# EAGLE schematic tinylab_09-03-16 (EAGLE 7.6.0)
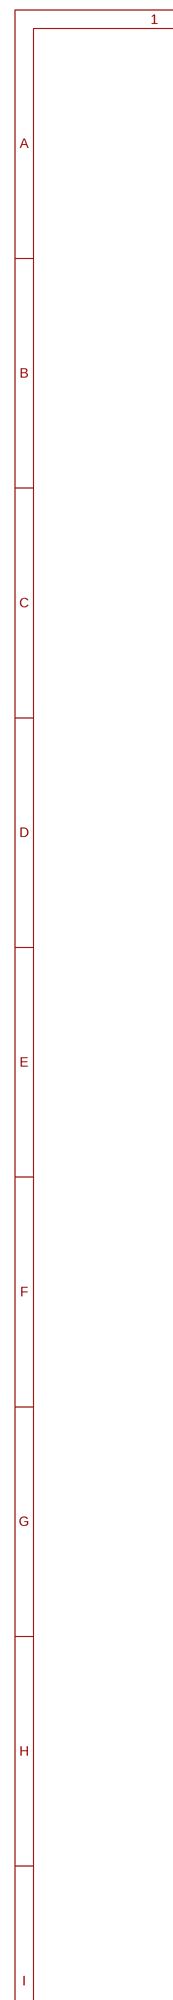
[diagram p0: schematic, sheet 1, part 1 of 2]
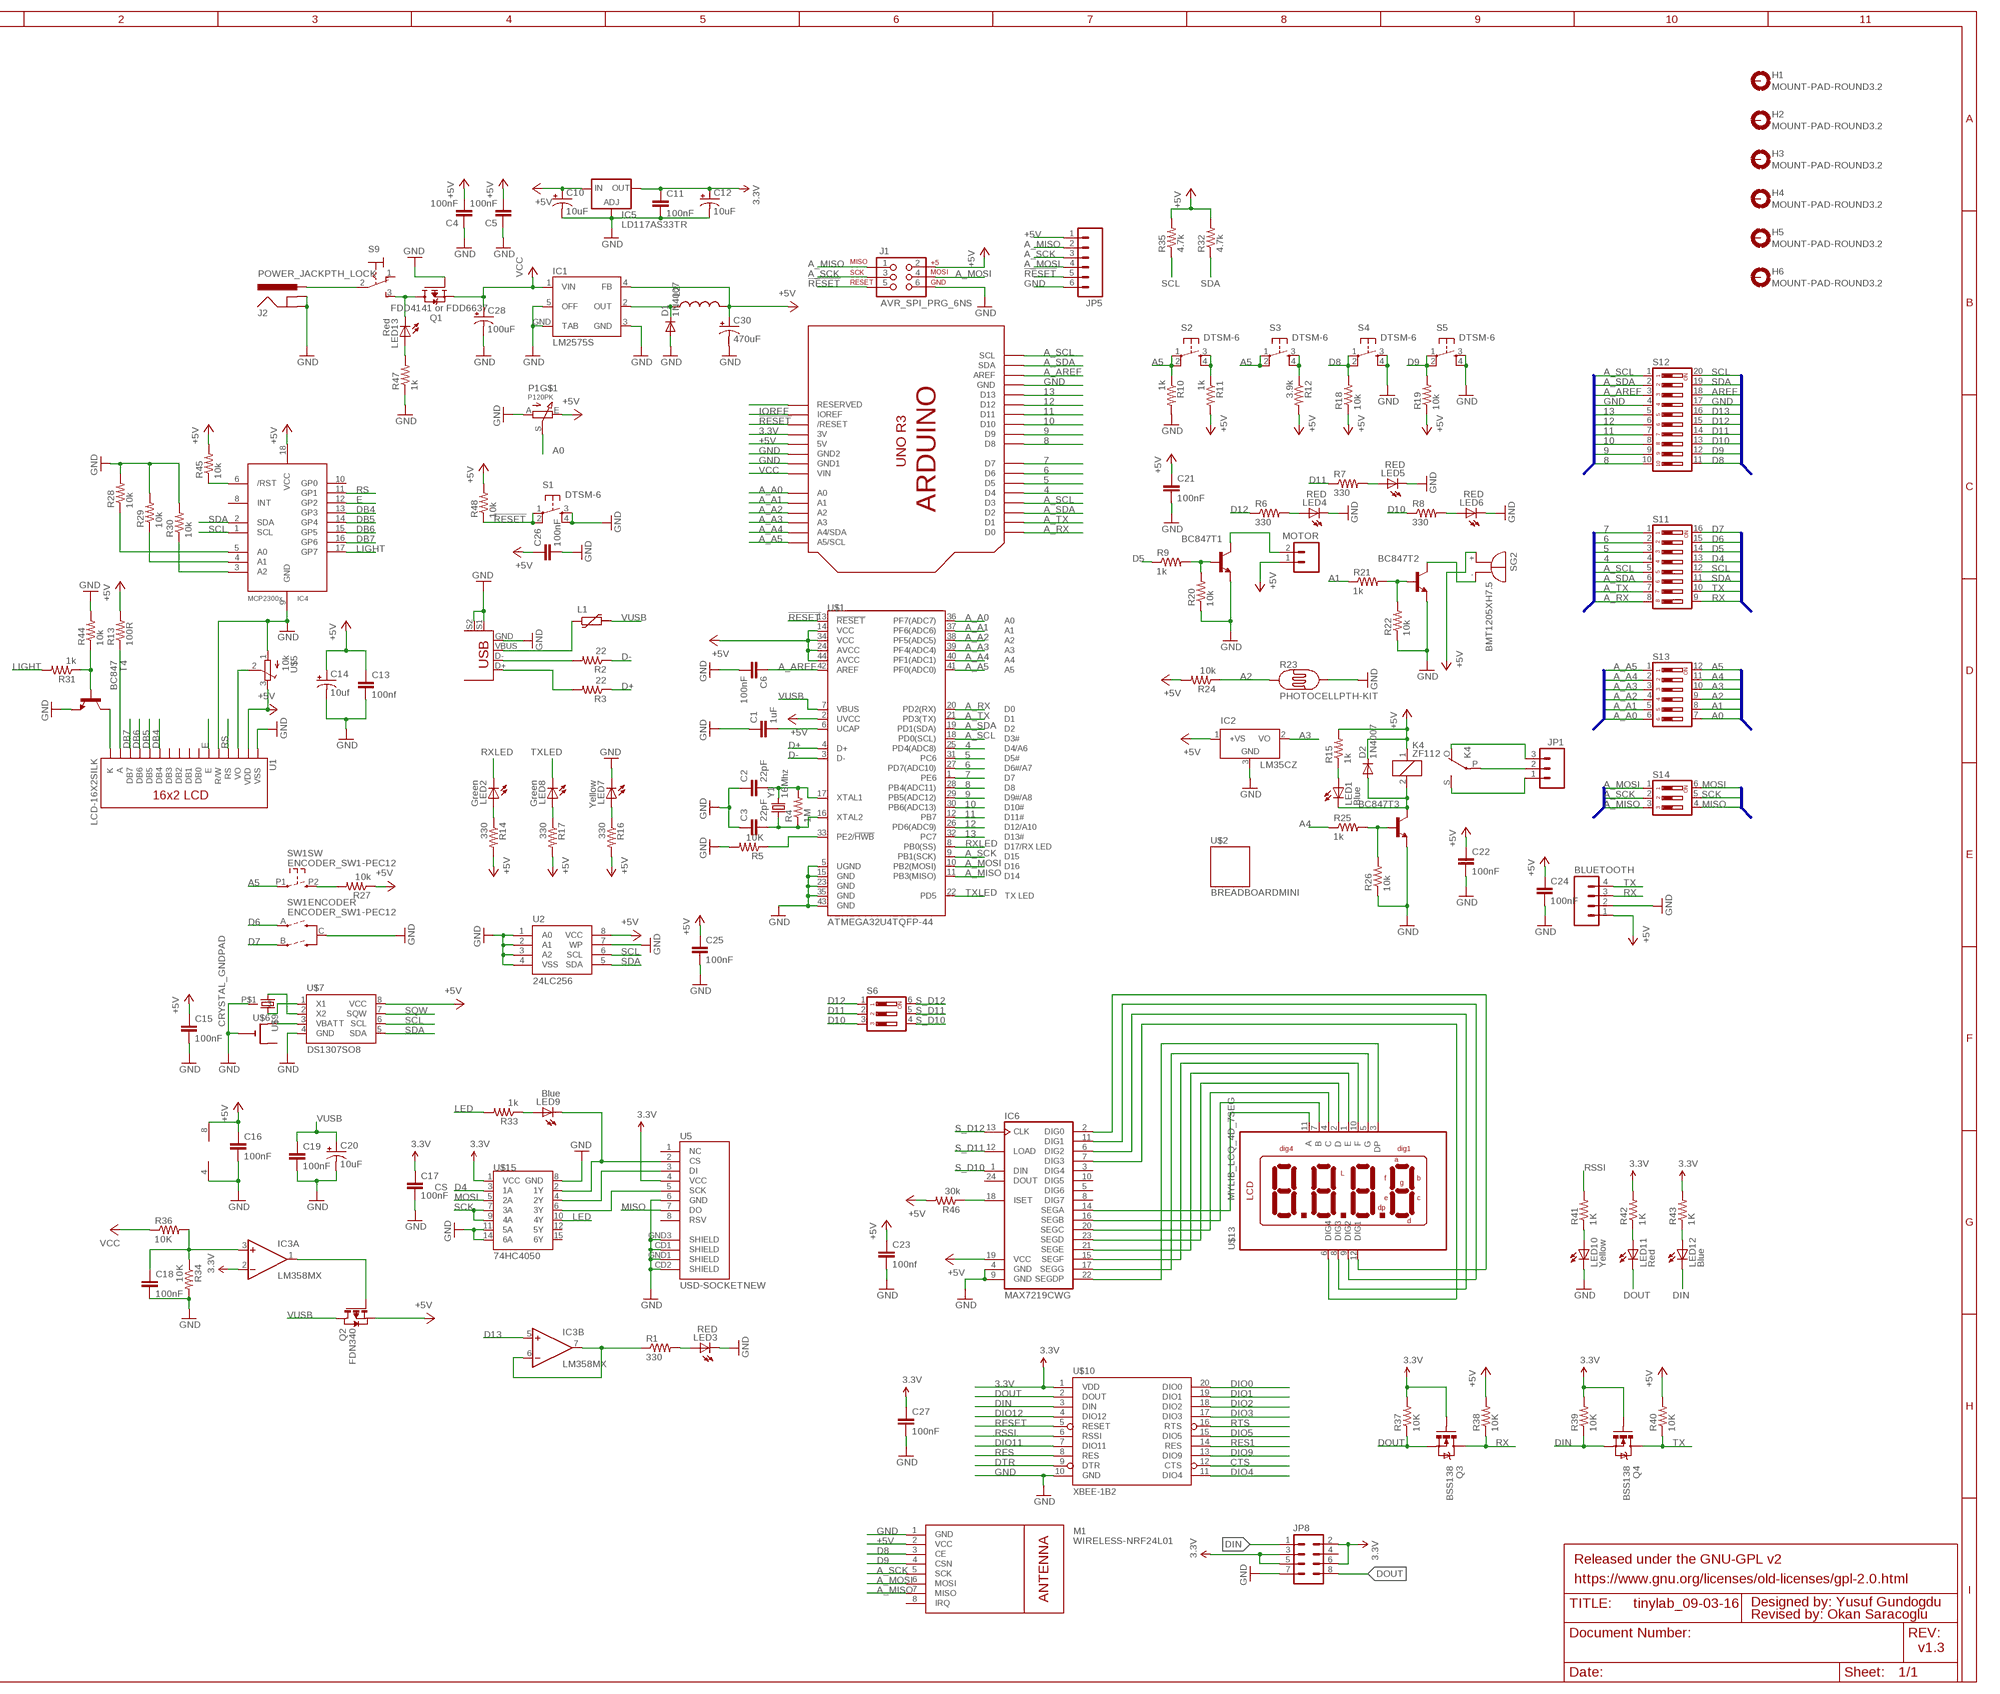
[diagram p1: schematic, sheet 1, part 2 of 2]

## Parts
BLUETOOTH  M04PTH  [1X04]
C1  1uF  CAP1206  [1206]
C2  22pF  CAP0805  [0805]
C3  22pF  CAP0805  [0805]
C4  100nF  CAP0805  [0805]
C5  100nF  CAP0805  [0805]
C6  100nF  CAP0805  [0805]
C10  10uF  CAP_POL1206  [EIA3216]
C11  100nF  CAP0805  [0805]
C12  10uF  CAP_POL1206  [EIA3216]
C13  100nf  CAP0805  [0805]
C14  10uf  CAP_POL1206  [EIA3216]
C15  100nF  CAP0805  [0805]
C16  100nF  CAP0805  [0805]
C17  100nF  CAP0805  [0805]
C18  100nF  CAP0805  [0805]
C19  100nF  CAP0805  [0805]
C20  10uF  CAP_POL1206  [EIA3216]
C21  100nF  CAP0805  [0805]
C22  100nF  CAP0805  [0805]
C23  100nf  CAP0805  [0805]
C24  100nF  CAP0805  [0805]
C25  100nF  CAP0805  [0805]
C26  100nF  CAP0805  [0805]
C27  100nF  CAP0805  [0805]
C28  100uF  CAP_POLF80  [NIPPON_F80]
C30  470uF  CAP_POLG  [PANASONIC_G]
D1  1N4007  DIODESMA-ALT  [SMA-DIODE_ALT]
D2  1N4007  DIODESMA-ALT  [SMA-DIODE_ALT]
H1  MOUNT-PAD-ROUND3.2  [3,2-PAD]
H2  MOUNT-PAD-ROUND3.2  [3,2-PAD]
H3  MOUNT-PAD-ROUND3.2  [3,2-PAD]
H4  MOUNT-PAD-ROUND3.2  [3,2-PAD]
H5  MOUNT-PAD-ROUND3.2  [3,2-PAD]
H6  MOUNT-PAD-ROUND3.2  [3,2-PAD]
IC1  LM2575S  [TO263-5]
IC2  LM35CZ  [TO92]
IC3  LM358MX  [SO08]
IC4  MCP2300X/SO  [SO18W]
IC5  LD117AS33TR  [SOT223]
IC6  MAX7219CWG  [SO24W]
J1  AVR_SPI_PRG_6NS  [2X3-NS]
J2  POWER_JACKPTH_LOCK  [POWER_JACK_PTH_LOCK]
JP1  M03-SCREW-5MM  [SCREWTERMINAL-5MM-3]
JP5  M06SIP  [1X06]
JP8  M04X2  [2X4]
K4  ZF112  [ZF112]
L1  FUSE_PTC-0805  [PTC0805]
L2  INDUCTORPWR  [CDRH125]
LED1  Blue  LEDCHIPLED_0805  [CHIPLED_0805]
LED2  Green  LEDCHIPLED_0805  [CHIPLED_0805]
LED3  RED  LED5MM  [LED5MM]
LED4  RED  LED5MM  [LED5MM]
LED5  RED  LED5MM  [LED5MM]
LED6  RED  LED5MM  [LED5MM]
LED7  Yellow  LEDCHIPLED_0805  [CHIPLED_0805]
LED8  Green  LEDCHIPLED_0805  [CHIPLED_0805]
LED9  Blue  LEDCHIPLED_0805  [CHIPLED_0805]
LED10  Yellow  LEDCHIPLED_0805  [CHIPLED_0805]
LED11  Red  LEDCHIPLED_0805  [CHIPLED_0805]
LED12  Blue  LEDCHIPLED_0805  [CHIPLED_0805]
LED13  Red  LEDCHIPLED_0805  [CHIPLED_0805]
M1  WIRELESS-NRF24L01  [WIRELESS-NRF24L01]
MOTOR  M025MM  [SCREWTERMINAL-5MM-2]
P1  P120PK  [P120PK]
Q1  FDD4141 or FDD6637  FDD4141TO252  [TO252]
Q2  FDN340  PMOSSOT23  [SOT-23]
Q3  BSS138  MOSFET-NCHANNELSMD  [SOT23-3]
Q4  BSS138  MOSFET-NCHANNELSMD  [SOT23-3]
R1  330  RESISTOR0805-RES  [0805]
R2  22  RESISTOR0805-RES  [0805]
R3  22  RESISTOR0805-RES  [0805]
R4  1M  RESISTOR0805-RES  [0805]
R5  10K  RESISTOR0805-RES  [0805]
R6  330  RESISTOR0805-RES  [0805]
R7  330  RESISTOR0805-RES  [0805]
R8  330  RESISTOR0805-RES  [0805]
R9  1k  RESISTOR0805-RES  [0805]
R10  1k  RESISTOR0805-RES  [0805]
R11  1k  RESISTOR0805-RES  [0805]
R12  3.9k  RESISTOR0805-RES  [0805]
R13  100R  RESISTOR0805-RES  [0805]
R14  330  RESISTOR0805-RES  [0805]
R15  1k  RESISTOR0805-RES  [0805]
R16  330  RESISTOR0805-RES  [0805]
R17  330  RESISTOR0805-RES  [0805]
R18  10k  RESISTOR0805-RES  [0805]
R19  10k  RESISTOR0805-RES  [0805]
R20  10k  RESISTOR0805-RES  [0805]
R21  1k  RESISTOR0805-RES  [0805]
R22  10k  RESISTOR0805-RES  [0805]
R23  PHOTOCELLPTH-KIT  [PHOTOCELL-KIT]
R24  10k  RESISTOR0805-RES  [0805]
R25  1k  RESISTOR0805-RES  [0805]
R26  10k  RESISTOR0805-RES  [0805]
R27  10k  RESISTOR0805-RES  [0805]
R28  10k  RESISTOR0805-RES  [0805]
R29  10k  RESISTOR0805-RES  [0805]
R30  10k  RESISTOR0805-RES  [0805]
R31  1k  RESISTOR0805-RES  [0805]
R32  4.7k  RESISTOR0805-RES  [0805]
R33  1k  RESISTOR0805-RES  [0805]
R34  10K  RESISTOR0805-RES  [0805]
R35  4.7k  RESISTOR0805-RES  [0805]
R36  10K  RESISTOR0805-RES  [0805]
R37  10K  RESISTOR0805-RES  [0805]
R38  10K  RESISTOR0805-RES  [0805]
R39  10K  RESISTOR0805-RES  [0805]
R40  10K  RESISTOR0805-RES  [0805]
R41  1K  RESISTOR0805-RES  [0805]
R42  1K  RESISTOR0805-RES  [0805]
R43  1K  RESISTOR0805-RES  [0805]
R44  10k  RESISTOR0805-RES  [0805]
R45  10k  RESISTOR0805-RES  [0805]
R46  30k  RESISTOR0805-RES  [0805]
R47  1k  RESISTOR0805-RES  [0805]
R48  10k  RESISTOR0805-RES  [0805]
S1  DTSM-6  [DTSM-6]
S2  DTSM-6  [DTSM-6]
S3  DTSM-6  [DTSM-6]
S4  DTSM-6  [DTSM-6]
S5  DTSM-6  [DTSM-6]
S6  DIP03YL  [DIP03YL]
S9  M9040P  [M9040P]
S11  DIP08YL  [DIP08YL]
S12  DIP10YL  [DIP10YL]
S13  DIP06YL  [DIP06YL]
S14  DIP03YL  [DIP03YL]
SG2  BMT1205XH7.5  [BMT1205XH7.5]
SW1  ENCODER_SW1-PEC12  [PEC12_INCREMENTAL_ENCODER]
T1  BC847  MMBT2222ALT1-NPN-SOT23-BEC  [SOT23-BEC]
T2  BC847  MMBT2222ALT1-NPN-SOT23-BEC  [SOT23-BEC]
T3  BC847  MMBT2222ALT1-NPN-SOT23-BEC  [SOT23-BEC]
T4  BC847  MMBT2222ALT1-NPN-SOT23-BEC  [SOT23-BEC]
U1  LCD-16X2SILK  [LCD-16X2]
U2  24LC256  EEPROM-I2CSMD  [SO08]
U5  USD-SOCKETNEW  [MICRO-SD-SOCKET-PP]
U$1  ATMEGA32U4TQFP-44  [TQFP44]
U$2  BREADBOARDMINI  [BREADBOARD-MINI]
U$3  USB+SHIELD  [USB-B-PTH]
U$4  UNO_R3  [UNO_R3]
U$5  10k  TRIMPOTTC33X  [TC33X]
U$6  CR1220SMT  [CR1220-SMD]
U$7  DS1307SO8  [SO08]
U$9  CRYSTAL_GNDPAD  [TC38H_GNDPAD]
U$10  XBEE-1B2  [XBEE-SILK]
U$13  MYLIB_LCQ_4D_7SEG  [MYLIB_LDQ_4D_7SEG]
U$15  74HC4050  HEX_CONVERTER  [SO016]
Y1  16Mhz  CRYSTAL5X3  [CRYSTAL-SMD-5X3]

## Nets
3.3V: C11.1 C12.A(+) C17.1 C27.1 IC3.2(A:-IN) IC5.4(OUT) JP8.2 JP8.3 JP8.5 JP8.6 Q3.1(G) Q4.1(G) R37.2 R39.2 R42.2 R43.2 U5.4(VCC) U$4.3V U$10.1(VDD) U$15.1(VCC)
4: S11.4 U$1.25(PD4(ADC8)) U$4.D4
5: S11.3 U$1.31(PC6) U$4.D5
6: S11.2 U$1.27(PD7(ADC10)) U$4.D6
7: S11.1 U$1.1(PE6) U$4.D7
8: S12.10 U$1.28(PB4(ADC11)) U$4.D8
9: S12.9 U$1.29(PB5(ADC12)) U$4.D9
10: S12.8 U$1.30(PB6(ADC13)) U$4.D10
11: S12.7 U$1.12(PB7) U$4.D11
12: S12.6 U$1.26(PD6(ADC9)) U$4.D12
13: S12.5 U$1.32(PC7) U$4.D13
!RESET: J1.5 JP5.5 R48.1 S1.1 S1.2 U$1.13(!RESET) U$4.RESET(/RESET)
+5V: BLUETOOTH.1 C4.2 C5.2 C10.A(+) C13.1 C14.A(+) C15.1 C16.1 C21.1 C22.1 C23.1 C24.1 C25.1 C26.1 C30.+ D2.C IC1.4(FB) IC2.1(+VS) IC3.8(P:V+) IC4.18(VCC) IC5.3(IN) IC6.19(VCC) J1.2 JP5.1 K4.1 L2.2 M1.2(VCC) MOTOR.1 P1.E Q2.2(S) R11.2 R12.2 R13.2 R14.2 R15.2 R16.2 R17.2 R18.1 R19.1 R24.2 R27.1 R32.2 R35.2 R38.2 R40.2 R45.2 R46.2 R48.2 SG2.+ U1.2(VDD) U2.8(VCC) U$1.2(UVCC) U$1.14(VCC) U$1.24(AVCC) U$1.34(VCC) U$1.44(AVCC) U$4.5V U$5.3(E) U$7.8(VCC)
A0: P1.S S13.7
A1: R21.1 S13.8
A2: R23.1 R24.1 S13.9
A3: IC2.2(VO) S13.10
A4: R25.1 S13.11
A5: R10.1 S2.1 S2.2 S3.1 S3.2 S13.12 SW1.P1
A_A0: S13.6 U$1.36(PF7(ADC7)) U$4.A0
A_A1: S13.5 U$1.37(PF6(ADC6)) U$4.A1
A_A2: S13.4 U$1.38(PF5(ADC5)) U$4.A2
A_A3: S13.3 U$1.39(PF4(ADC4)) U$4.A3
A_A4: S13.2 U$1.40(PF1(ADC1)) U$4.A4(A4/SDA)
A_A5: S13.1 U$1.41(PF0(ADC0)) U$4.A5(A5/SCL)
A_AREF: C6.1 S12.3 U$1.42(AREF) U$4.AREF
A_MISO: J1.1 JP5.2 M1.7(MISO) S14.3 U$1.11(PB3(MISO))
A_MOSI: J1.4 JP5.4 M1.6(MOSI) S14.1 U$1.10(PB2(MOSI))
A_RX: S11.8 U$1.20(PD2(RX)) U$4.D0
A_SCK: J1.3 JP5.3 M1.5(SCK) S14.2 U$1.9(PB1(SCK))
A_SCL: S11.5 S12.1 U$1.18(PD0(SCL)) U$4.D3 U$4.SCL
A_SDA: S11.6 S12.2 U$1.19(PD1(SDA)) U$4.D2 U$4.SDA
A_TX: S11.7 U$1.21(PD3(TX)) U$4.D1
AREF: S12.18
CTS: U$10.12(CTS)
D4: S11.13 U$15.3(1A)
D5: R9.1 S11.14
D6: S11.15 SW1.A(ENCODER:A)
D7: S11.16 SW1.B(ENCODER:B)
D8: M1.3(CE) R18.2 S4.1 S4.2 S12.11
D9: M1.4(CSN) R19.2 S5.1 S5.2 S12.12
D10: R8.1 S6.3 S12.13
D11: R7.1 S6.2 S12.14
D12: R6.1 S6.1 S12.15
D13: IC3.5(B:+IN) S12.16
D+: R3.1 U$1.4(D+)
D-: R2.1 U$1.3(D-)
DB4: IC4.13(GP3) U1.11(DB4)
DB5: IC4.14(GP4) U1.12(DB5)
DB6: IC4.15(GP5) U1.13(DB6)
DB7: IC4.16(GP6) U1.14(DB7)
DIN: JP8.1 LED12.C Q4.2(S) R39.1 U$10.3(DIN)
DIO0: U$10.20(DIO0)
DIO1: U$10.19(DIO1)
DIO2: U$10.18(DIO2)
DIO3: U$10.17(DIO3)
DIO4: U$10.11(DIO4)
DIO5: U$10.15(DIO5)
DIO9: U$10.13(DIO9)
DIO11: U$10.7(DIO11)
DIO12: U$10.4(DIO12)
DOUT: JP8.8 LED11.C Q3.2(S) R37.1 U$10.2(DOUT)
DTR: U$10.9(DTR)
E: IC4.12(GP2) U1.6(E)
GND: BLUETOOTH.2 C1.1 C2.1 C3.1 C4.1 C5.1 C6.2 C10.C(-) C11.2 C12.C(-) C13.2 C14.C(-) C15.2 C16.2 C17.2 C18.2 C19.2 C20.C(-) C21.2 C22.2 C23.2 C24.2 C25.2 C26.2 C27.2 C28.- C30.- D1.A IC1.3(GND) IC1.5(OFF) IC1.GND(TAB) IC2.3(GND) IC3.4(P:V-) IC4.9(GND) IC5.1(ADJ) IC6.4(GND) IC6.9(GND) J1.6 J2.GND J2.GNDBREAK JP5.6 JP8.7 LED3.K(C) LED4.K(C) LED5.K(C) LED6.K(C) LED7.C LED10.C M1.1(GND) P1.A Q1.1(G) R5.2 R10.2 R20.1 R22.1 R23.2 R26.1 R28.2 R29.2 R30.2 R34.2 R44.2 R47.1 S1.3 S1.4 S4.3 S4.4 S5.3 S5.4 S12.4 S12.17 SW1.C(ENCODER:C) T1.E T2.E T3.E T4.E U1.1(VSS) U1.5(R/W) U2.1(A0) U2.2(A1) U2.3(A2) U2.4(VSS) U2.7(WP) U5.6(GND) U5.CD1(SHIELD) U5.CD2(SHIELD) U5.GND1(SHIELD) U5.GND3(SHIELD) U$1.5(UGND) U$1.15(GND) U$1.23(GND) U$1.35(GND) U$1.43(GND) U$3.GND U$3.S1 U$3.S2 U$4.GND U$4.GND1 U$4.GND2 U$5.1(A) U$6.- U$7.4(GND) U$9.P$1 U$10.10(GND) U$15.8(GND) U$15.11(5A) U$15.14(6A)
IOREF: U$4.IOREF
LED: R33.2 U$15.10(4Y)
LIGHT: IC4.17(GP7) R31.2
MISO: S14.4 U5.7(DO)
MOSI: S14.6 U$15.5(2A)
N$1: R2.2 U$3.D-
N$2: R3.2 U$3.D+
N$3: LED3.A R1.2
N$4: C1.2 U$1.6(UCAP)
N$5: R11.1 S2.3 S2.4
N$6: C3.2 R4.1 U$1.16(XTAL2) Y1.1
N$7: C2.2 R4.2 U$1.17(XTAL1) Y1.3
N$8: R21.2 R22.2 T2.B
N$9: R5.1 U$1.33(PE2/!HWB)
N$10: D1.C IC1.2(OUT) L2.1
N$11: R12.1 S3.3 S3.4
N$12: R9.2 R20.2 T1.B
N$13: LED4.A R6.2
N$14: JP1.3 K4.O(2:O)
N$15: LED5.A R7.2
N$16: MOTOR.2 T1.C
N$17: LED6.A R8.2
N$18: SG2.- T2.C
N$19: LED1.A R15.1
N$20: R25.2 R26.2 T3.B
N$21: D2.A K4.2 LED1.C T3.C
N$22: LED2.A R14.1
N$23: LED8.A R17.1
N$24: JP1.2 K4.P(2:P)
N$25: JP1.1 K4.S(2:S)
N$26: J2.PWR S9.2(P)
N$27: LED13.C Q1.3(D) S9.3(S)
N$28: U$4.RESERVED
N$29: IC4.5(A0) R28.1
N$30: IC4.4(A1) R29.1
N$31: IC4.3(A2) R30.1
N$32: R27.2 SW1.P2
N$33: R31.1 R44.1 T4.B
N$34: U1.3(VO) U$5.2(S)
N$35: T4.C U1.16(K)
N$36: U$7.2(X2) U$9.1
N$37: U$6.+$1(+) U$7.3(VBATT)
N$38: IC6.14(SEGA) U$13.11(A)
N$39: U5.3(DI) U$15.4(2Y)
N$40: U5.5(SCK) U$15.6(3Y)
N$41: U$7.1(X1) U$9.2
N$42: LED9.A R33.1
N$43: LED9.C U5.2(CS) U$15.2(1Y)
N$44: L1.1 U$3.VBUS
N$45: C18.1 IC3.3(A:+IN) R34.1 R36.2
N$46: LED10.A R41.1
N$47: IC3.1(A:OUT) Q2.3(G)
N$48: IC3.6(B:-IN) IC3.7(B:OUT) R1.1
N$49: LED11.A R42.1
N$50: LED12.A R43.1
N$51: LED13.A R47.2
N$52: IC4.6(/RST) R45.1
N$53: IC6.18(ISET) R46.1
N$54: IC6.16(SEGB) U$13.7(B)
N$55: IC6.20(SEGC) U$13.4(C)
N$56: IC6.23(SEGD) U$13.2(D)
N$57: IC6.21(SEGE) U$13.1(E)
N$58: IC6.15(SEGF) U$13.10(F)
N$59: IC6.17(SEGG) U$13.5(G)
N$60: IC6.22(SEGDP) U$13.3(DP)
N$61: IC6.7(DIG3) U$13.6(DIG4)
N$62: IC6.6(DIG2) U$13.8(DIG3)
N$63: IC6.11(DIG1) U$13.9(DIG2)
N$64: IC6.2(DIG0) U$13.12(DIG1)
N$65: R13.1 U1.15(A)
N$119: LED7.A R16.1
RES: U$10.8(RES)
RES1: U$10.14(RES)
RESET: U$10.5(RESET)
RS: IC4.11(GP1) U1.4(RS)
RSSI: R41.2 U$10.6(RSSI)
RTS: U$10.16(RTS)
RX: BLUETOOTH.3 Q3.3(D) R38.1 S11.9
RXLED: LED2.C U$1.8(PB0(SS))
S_D10: IC6.1(DIN) S6.4
S_D11: IC6.12(LOAD) S6.5
S_D12: IC6.13(CLK) S6.6
SCK: S14.5 U$15.7(3A) U$15.9(4A)
SCL: IC4.1(SCL) R35.1 S11.12 S12.20 U2.6(SCL) U$7.6(SCL)
SDA: IC4.2(SDA) R32.1 S11.11 S12.19 U2.5(SDA) U$7.5(SDA)
SQW: U$7.7(SQW)
TX: BLUETOOTH.4 Q4.3(D) R40.1 S11.10
TXLED: LED8.C U$1.22(PD5)
VCC: C28.+ IC1.1(VIN) Q1.2(S) R36.1 U$4.VIN
VUSB: C19.1 C20.A(+) L1.2 Q2.1(D) U$1.7(VBUS)
Unconnected: H1.B3,2(MOUNT) H2.B3,2(MOUNT) H3.B3,2(MOUNT) H4.B3,2(MOUNT) H5.B3,2(MOUNT) H6.B3,2(MOUNT) IC4.8(INT) IC4.10(GP0) IC6.3(DIG4) IC6.5(DIG6) IC6.8(DIG7) IC6.10(DIG5) IC6.24(DOUT) JP8.4 M1.8(IRQ) P1.M1(GND) P1.M2(GND) S9.1(O) U1.7(DB0) U1.8(DB1) U1.9(DB2) U1.10(DB3) U5.1(NC) U5.8(RSV) U$6.+$2(+1) U$15.12(5Y) U$15.15(6Y)

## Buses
SCL,SDA,AREF,GND,D13,D12,D11,D10,D9,D8
D7,D6,D5,D4,SCL,SDA,TX,RX
A0,A1,A2,A3,A4,A5
A_SCL,A_SDA,A_AREF,GND,13,12,11,10,9,8
7,6,5,4,A_SCL,A_SDA,A_TX,A_RX
A_A0,A_A1,A_A2,A_A3,A_A4,A_A5
MOSI,SCK,MISO
A_MOSI,A_SCK,A_MISO

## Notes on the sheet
- CS
- Released under the GNU-GPL v2
- https://www.gnu.org/licenses/old-licenses/gpl-2.0.html
- Designed by: Yusuf Gundogdu
- Revised by: Okan Saracoglu
- v1.3

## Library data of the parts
BLUETOOTH = SparkFun:M04: Header 4 Standard 4-pin 0.1" header. Use with straight break away headers (SKU : PRT-00116), right angle break away headers (PRT-00553), swiss pins (PRT-00743), machine pins (PRT-00117), and female headers (PRT-00115). Molex polarized connector foot print use with SKU : PRT-08231 with associated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
C1-C6 C11 C13 C15-C19 C21-C27 = SparkFun:CAP: Capacitor
C10 C12 C14 C20 C28 C30 = SparkFun:CAP_POL: Capacitor Polarized
D1 D2 = SparkFun:DIODE: Diode
H1-H6 = holes:MOUNT-PAD-ROUND: MOUNTING PAD, round
IC1 = v-reg-3:LM2575: National Semiconductor 1.0A "Simple Switcher"(c) 52kHz, Vout 1.23-37V (HV: 57V), Vin 40V (HV: 60V), 50µA standby current
IC2 = lm35:LM35: Single-Supply Centigrade Temperature Sensor Vout = (10mV/°C x Temp °C) +5mmmV Source: http://www.national.com/ds/LM/LM35.pdf
IC3 = linear:LM358: OP AMP also LM158; LM258; LM2904 Source: http://cache.national.com/ds/LM/LM158.pdf
IC4 = adafruit:MCP2300X: MCP23008 Inexpensive i2c i/o expander - 8 general purpose i/o pins with optional pullups
IC5 = v-reg:LD117A?*: Low drop fixed and adjustable positive voltage regulators 1 A Source: http://www.st.com/stonline/products/literature/ds/7194/ld1117axx.pdf
IC6 = maxim-10:MAX7219*: Serially Interfaced, 8-Digit LED Display Drivers
J1 = SparkFun:AVR_SPI_PRG_6: AVR ISP 6 Pin This is the reduced ISP connector for AVR programming. Common on Arduino. This footprint will take up less PCB space and can be used with a 10-pin to 6-pin adapter such as SKU: BOB-08508
J2 = SparkFun:POWER_JACK: Power Jack This is the standard 5.5mm barrel jack for power. The PTH is the most common, proven, reliable, footprint. All others are experimental. The Slot footprint only works if the mill layer is transmitted to the PCB fab house so be warned. Spark Fun Electronics SKU : PRT-00119. Mating wall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
JP1 = SparkFun:M03: Header 3 Standard 3-pin 0.1" header. Use with straight break away headers (SKU : PRT-00116), right angle break away headers (PRT-00553), swiss pins (PRT-00743), machine pins (PRT-00117), and female headers (PRT-00115). Molex polarized connector foot print use with SKU : PRT-08232 with associated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
JP5 = SparkFun:M06: Header 6 Standard 6-pin 0.1" header. Use with straight break away headers (SKU : PRT-00116), right angle break away headers (PRT-00553), swiss pins (PRT-00743), machine pins (PRT-00117), and female headers (PRT-00115). Molex polarized connector foot print use with SKU : PRT-08094 with associated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
JP8 = SparkFun-Connectors:M04X2: .1" header, two rows of four.
K4 = relay:ZF112: RELAY 1 x switch; OC_FARNELL: unknown; OC_NEWARK: unknown
L1 = dp_devices:FUSE_PTC: Resettable PTC
L2 = SparkFun:INDUCTOR: Inductors
LED1 LED2 LED7-LED13 = led:LED: LED
LED3-LED6 = SparkFun:LED: LEDs
M1 = diy-modules:WIRELESS-NRF24L01: 2.4 GHz Wireless Module based on NRF24L01 chip
MOTOR = SparkFun-Connectors:M02: Standard 2-pin 0.1" header. Use with; STOREFRONT_ID: PRT-08432
P1 = pot-tt_electronics:P120PK
Q1 = transistor-fet:FDD4141: P-Channel PowerTrench® MOSFET Source: FDD4141.pdf
Q2 = zetex:PMOSSOT23: MOS FET; OC_FARNELL: unknown; OC_NEWARK: unknown
Q3 Q4 = SparkFun:MOSFET-NCHANNEL
R1-R22 R24-R48 = SparkFun:RESISTOR: Resistor
R23 = SparkFun:PHOTOCELL: Photocell Also known as a CdS photoresistor. This is a low cost way to detect light levels. Resistance decreases with more incoming light. SparkFun SKU: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
S1-S5 = switch-tact:DTSM-6
S6 S14 = switch-dil:DIP03YL: DIL/CODE SWITCH; OC_FARNELL: unknown; OC_NEWARK: unknown
S9 = switch:M9040P: TOGGLE SWITCH Marquardt
S11 = switch-dil:DIP08YL: DIL/CODE SWITCH; OC_FARNELL: unknown; OC_NEWARK: unknown
S12 = switch-dil:DIP10YL: DIL/CODE SWITCH; OC_FARNELL: unknown; OC_NEWARK: unknown
S13 = switch-dil:DIP06YL: DIL/CODE SWITCH; OC_FARNELL: unknown; OC_NEWARK: unknown
SG2 = buzzer:BMT1205XH7.5: MAGNETIC TRANSDUCER; OC_FARNELL: unknown; OC_NEWARK: unknown
SW1 = dp_devices:ENCODER_SW1: Incremental Encoder with push switch
T1-T4 = transistor:*-NPN-: NPN Transistror BF959 corrected 2008.03.06
U1 = SparkFun:LCD-16X2
U2 = SparkFun-DigitalIC:EEPROM-I2C: I2C EEPROM chips, 24LC256 (and others)
U5 = SparkFun:USD-SOCKET: microSD Socket Push-push type uSD socket. Schematic element and footprint production proven. Spark Fun Electronics SKU : PRT-00127. tDoc lines correctly indicate media card edge positions when inserting (unlocked, locked, depressed).
U$1 = SparkFun-DigitalIC:ATMEGA32U4: Atmel 44-pin 8-bit Microcontroller with 32KBytes of ISP Flash and USB Controller
U$2 = SparkFun:BREADBOARD: Breadboard Mini Self Adhesive
U$3 = SparkFun:USB+SHIELD: USB+Shield USB connector with shield pins connectable
U$4 = UNO_R3:UNO_R3
U$5 = adafruit:TRIMPOT: SMT trimmer potentiometer part number TC33X http://www.ladyada.net/library/eagle
U$6 = adafruit:CR1220: CR1216/CR1220/CR1225 12mm 3V lithium coin cell Great for battery packup. Both SMT and THM holders. Note the THM package has the ground pads on both sides of the PCB so that the masks are the same - this reduces the cost
U$7 = SparkFun:DS1307
U$9 = crystal:CRYSTAL_GNDPAD
U$10 = SparkFun:XBEE-1
U$13 = 4_Digit_DIsplay:MYLIB_LCQ_4D_7SEG
U$15 = SparkFun:HEX_CONVERTER
Y1 = SparkFun:CRYSTAL: Crystals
